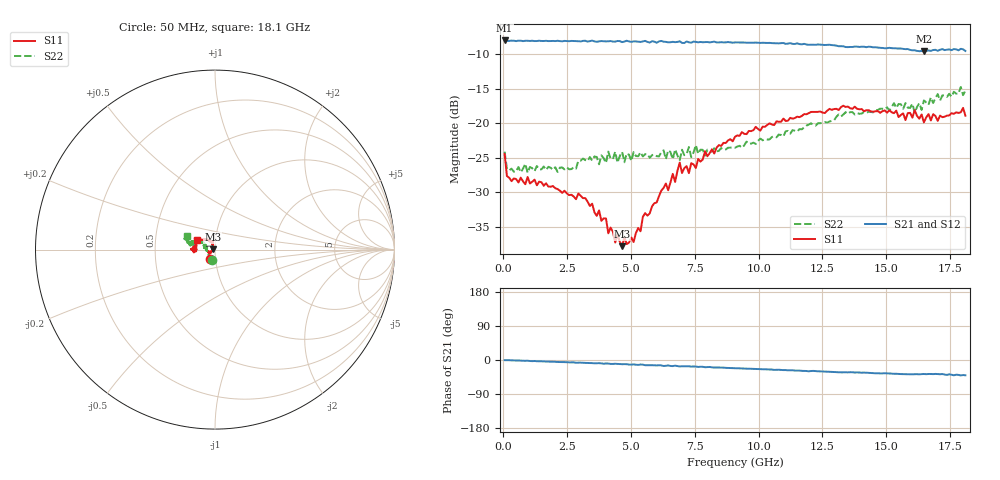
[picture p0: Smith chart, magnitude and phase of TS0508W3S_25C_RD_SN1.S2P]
! Network Analyzer HP8720D.06.14 Serial No. US36140669
! 17 Jun 2005  07:38:03
! Frequency  S11  S21  S12  S22
# HZ  S  DB R 50
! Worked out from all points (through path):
!   201 points, 50 MHz to 18.1 GHz, reference 50 ohm
!   highest |S21| = -8.05 dB at 50 MHz (marker M1); lowest = -9.6 dB at 16.48 GHz (marker M2)
!   group delay of S21, straight-line fit = 6.41 ps
!   lowest |S11| = -37.8 dB at 4.653 GHz (marker M3), VSWR 1.03, Z = 48.8 + j0.254 ohm
!   |S11| at or under -10 dB: start of sweep to end of sweep
!   |S22| runs from -27.2 to -14.8 dB; largest |S21 - S12| = 0.0095
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5e7  -24.46 -119.0  -8.05 -0.4  -8.08 0.1  -24.13 -106.6
1.4025e8  -27.66 -141.9  -8.10 -0.4  -8.09 -0.3  -26.55 -147.7
3.2075e8  -28.41 -155.6  -8.07 -0.9  -8.09 -0.8  -26.59 -165.1
3.1185e9  -30.86 -151.0  -8.11 -7.4  -8.17 -7.5  -25.13 170.8
4.021e9  -33.80 -155.9  -8.19 -9.3  -8.26 -9.2  -25.78 167.1
4.382e9  -37.28 -171.7  -8.22 -9.9  -8.16 -10.3  -24.14 169.2
4.47225e9  -36.15 179.3  -8.12 -10.4  -8.19 -10.1  -25.74 172.0
4.65275e9  -37.81 168.3  -8.28 -11.1  -8.18 -10.8  -24.17 172.4
4.743e9  -36.52 168.4  -8.21 -10.9  -8.25 -10.9  -25.66 168.0
5.104e9  -37.21 146.3  -8.18 -11.6  -8.13 -11.8  -24.19 164.7
6.09675e9  -30.58 115.4  -8.19 -13.9  -8.14 -14.0  -24.83 164.3
6.63825e9  -27.35 115.2  -8.24 -16.1  -8.31 -15.7  -25.23 158.8
6.7285e9  -28.52 115.4  -8.30 -14.9  -8.37 -15.6  -23.80 159.3
6.909e9  -25.72 113.2  -8.16 -17.1  -8.30 -16.7  -25.38 156.2
7.27e9  -27.24 111.3  -8.32 -16.6  -8.32 -17.4  -23.45 158.6
7.36025e9  -25.80 109.3  -8.37 -17.4  -8.35 -16.9  -24.93 161.6
7.54075e9  -26.50 111.1  -8.25 -17.2  -8.18 -18.1  -23.18 160.8
9.075e9  -21.98 133.8  -8.33 -21.5  -8.33 -21.5  -23.57 151.3
1.21435e10  -18.39 172.2  -8.67 -28.7  -8.67 -28.9  -20.24 153.3
1.512175e10  -18.15 -177.5  -9.11 -35.4  -9.11 -35.1  -18.15 163.7
1.64755e10  -19.90 179.7  -9.64 -36.9  -9.57 -36.6  -16.72 162.7
1.81e10  -18.92 152.8  -9.57 -40.3  -9.57 -41.7  -15.30 154.4
